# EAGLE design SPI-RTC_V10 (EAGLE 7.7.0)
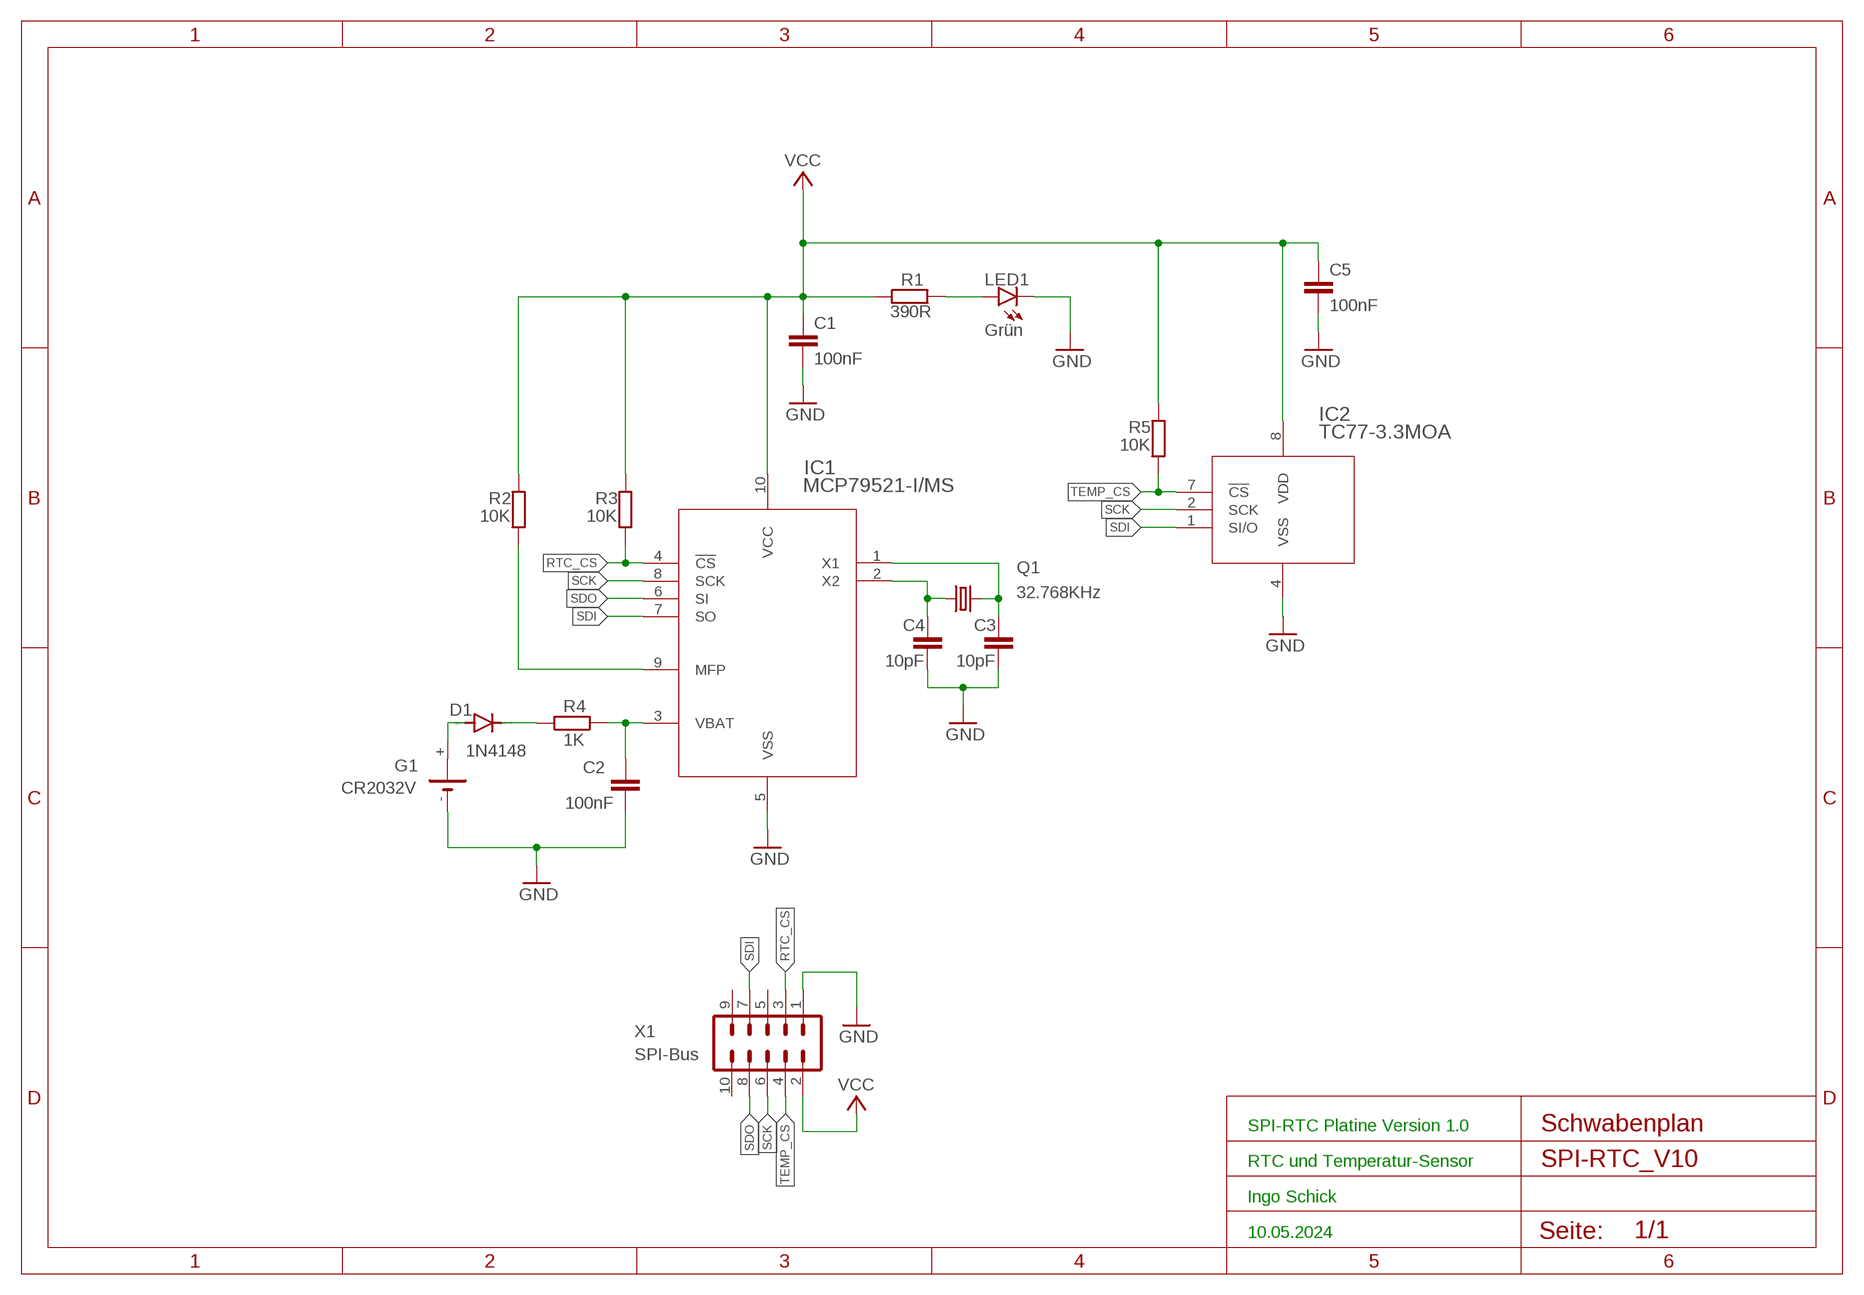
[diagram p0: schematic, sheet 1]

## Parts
C1  100nF  C-EU025-025X050  [C025-025X050]
C2  100nF  C-EU025-025X050  [C025-025X050]
C3  10pF  C-EU025-025X050  [C025-025X050]
C4  10pF  C-EU025-025X050  [C025-025X050]
C5  100nF  C-EU025-025X050  [C025-025X050]
D1  1N4148  1N4148DO35-7  [DO35-7]
G1  CR2032V  [CR2032V]
IC1  MCP79521-I/MS  [MSOP10]
IC2  TC77-3.3MOA  [SO-08]
LED1  Grün  LED3MM  [LED3MM]
Q1  32.768KHz  CRYSTALTC38H  [TC38H]
R1  390R  R-EU_0207/10  [0207/10]
R2  10K  R-EU_0207/10  [0207/10]
R3  10K  R-EU_0207/10  [0207/10]
R4  1K  R-EU_0207/10  [0207/10]
R5  10K  R-EU_0207/10  [0207/10]
X1  SPI-Bus  ML10  [ML10]

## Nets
BAT: D1.A G1.+
BAT_R: D1.C R4.2
GND: C1.2 C2.2 C3.2 C4.2 C5.2 G1.- IC1.5(VSS) IC2.4(VSS) LED1.K(C) X1.1
LED: LED1.A R1.2
MFP: IC1.9(MFP) R2.1
RTC_CS: IC1.4(!CS) R3.1 X1.3
SCK: IC1.8(SCK) IC2.2(SCK) X1.6
SDI: IC1.7(SO) IC2.1(SI/O) X1.7
SDO: IC1.6(SI) X1.8
TEMP_CS: IC2.7(!CS) R5.1 X1.4
VBAT: C2.1 IC1.3(VBAT) R4.1
VCC: C1.1 C5.1 IC1.10(VCC) IC2.8(VDD) R1.1 R2.2 R3.2 R5.2 X1.2
X1: C3.1 IC1.1(X1) Q1.2
X2: C4.1 IC1.2(X2) Q1.1
Unconnected: G1.+@1(+) X1.5 X1.9 X1.10

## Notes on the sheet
- SPI-RTC Platine Version 1.0
- RTC und Temperatur-Sensor
- Ingo Schick
- 10.05.2024

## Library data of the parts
C1-C5 = rcl:C-EU: CAPACITOR, European symbol; SPICEPREFIX: C
D1 = Schwabenplan:1N4148: 1N4148 -> Kleinsignal-Schaltdiode; FRITSCH: K-DI0001; HERSTELLER: 1N4148; MOUSER: 637-1N4148
G1 = Schwabenplan:CR2032V: Batteriehalter für CR2032; FRITSCH: K-BA0047; WUERTH: 79548211
IC1 = Schwabenplan_SPI:MCP79521: MCP79521-I/MS - SPI-Bus RTC-Baustein, EEPROM inkl. MAC-Adresse Produktinformationen: Datenblatt; HERSTELLER: MCP79521-I/MS; MOUSER: 579-MCP79521-I/MS
IC2 = Schwabenplan_SPI:TC77: TC77 - SPI-Bus Temperatur Sensor mit 13 Bit Auflösung Produktinformationen: Datenblatt; HERSTELLER: TC77-3.3MOA; MOUSER: 579-TC77-3.3MOA
LED1 = Schwabenplan_LED:LED: Schwabenplan LED
Q1 = Schwabenplan_Quarze:CRYSTAL: CRYSTAL; OC_FARNELL: unknown; OC_NEWARK: unknown
R1-R5 = rcl:R-EU_: RESISTOR, European symbol; SPICEPREFIX: R
X1 = Schwabenplan:ML10: IDE Wannenstecker 10 polig Würth: Datenblatt oder Harting: Datenblatt oder Reichelt: Datenblatt; FRITSCH: K-ST2236; HARTING: 09185106324; REICHELT: WSL 10G; WUERTH: 61201021621

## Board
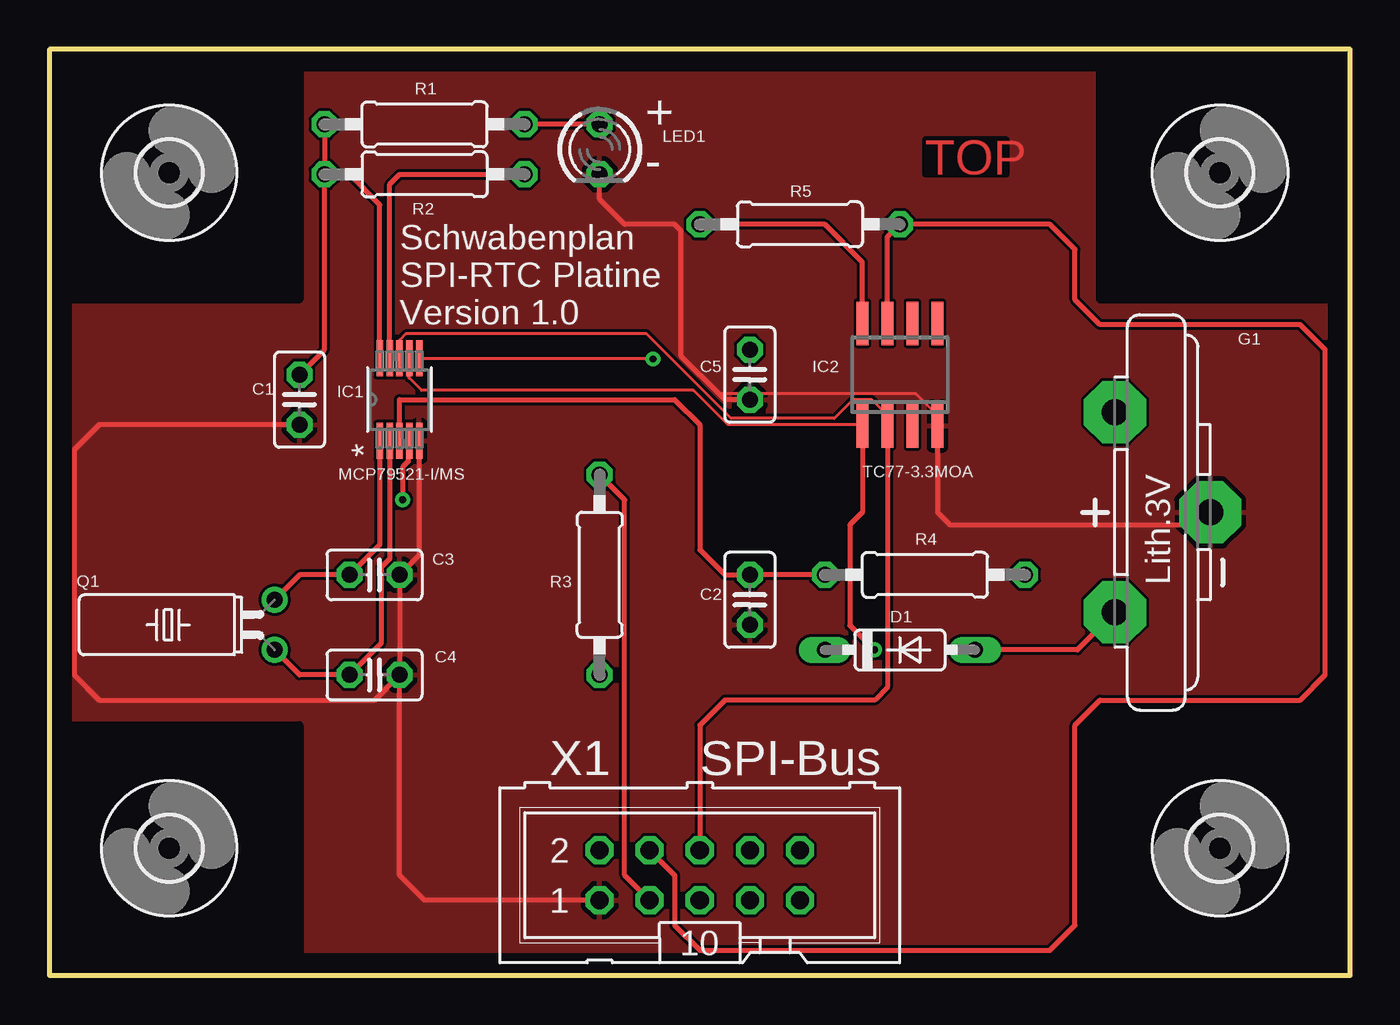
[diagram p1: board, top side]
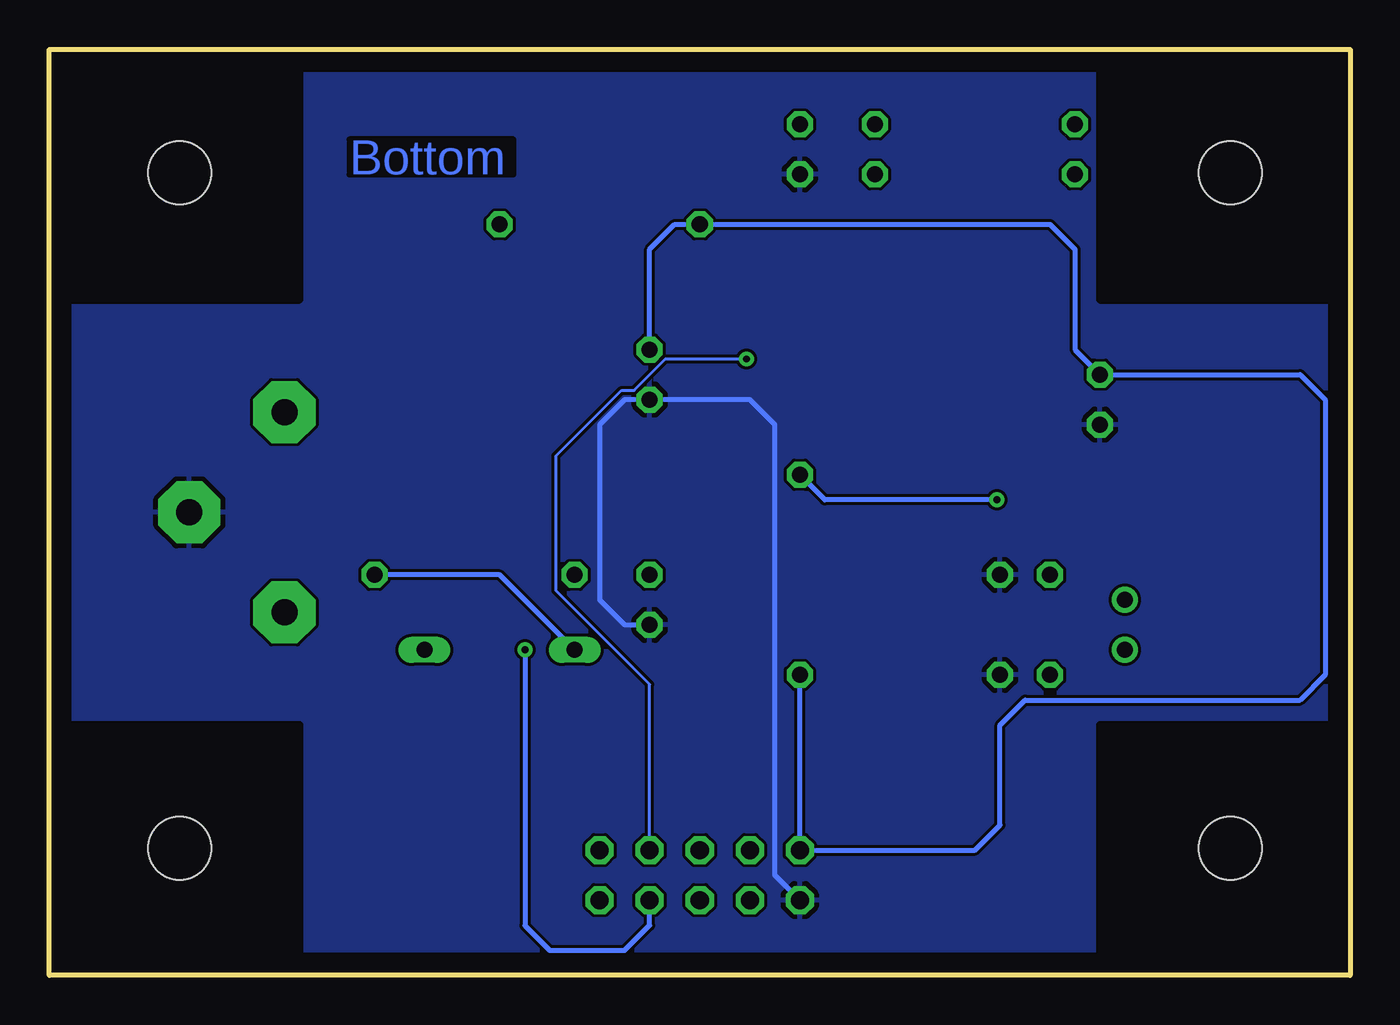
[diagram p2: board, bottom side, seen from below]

Size 66.04 x 46.99 mm. Coordinates in mm from the lower left corner, seen from the top.
Outline: 0,0 66.04,0 66.04,46.99 0,46.99 0,0
Copper layers (1*16): Top 0.035mm / dielectric 0.15mm / Bottom 0.035mm
Design rules "default": minimum track width 6mil, minimum drill 0.35mm, track to track 6mil, track to pad 6mil, pad to pad 6mil, via to via 6mil, smd to smd 6mil, copper to edge 40mil, drill to drill 6mil, minimum pad ring 10mil, minimum via ring 8mil, stop-mask expansion 4mil, vias tented up to drill 0mil, thermal gap 10mil
tRestrict: area 0,0 to 12.7,12.7; area 53.3,0 to 66,12.7; area 0,34.3 to 12.7,47; area 53.3,34.3 to 66,47
bRestrict: area 0,0 to 12.7,12.7; area 0,34.3 to 12.7,47; area 53.3,34.3 to 66,47; area 53.3,0 to 66,12.7

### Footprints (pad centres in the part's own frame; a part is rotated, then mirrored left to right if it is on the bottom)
C025-025X050 = drill 0.813 octagon: 1 -1.27,0; 2 1.27,0
DO35-7 = drill 0.813 long: A 3.81,0; C -3.81,0
CR2032V = drill 1.321 pad 3.15 octagon: + -2.54,-5.08; +@1 -2.54,5.08; - 2.286,0
MSOP10 = smd 1.829 x 0.33: 1 -2.095,1; 2 -2.095,0.5; 3 -2.095,0; 4 -2.095,-0.5; 5 -2.095,-1; 6 2.095,-1; 7 2.095,-0.5; 8 2.095,0; 9 2.095,0.5; 10 2.095,1
SO-08 = smd 0.6 x 2.2: 1 -1.905,-2.6; 2 -0.635,-2.6; 3 0.635,-2.6; 4 1.905,-2.6; 5 1.905,2.6; 6 0.635,2.6; 7 -0.635,2.6; 8 -1.905,2.6
LED3MM = drill 0.813 octagon: A -1.27,0; K 1.27,0
TC38H = drill 0.813: 1 -1.27,0; 2 1.27,0
0207/10 = drill 0.813 octagon: 1 -5.08,0; 2 5.08,0
3,2 = hole 3.2: 0,0
ML10 = drill 0.914 octagon: 1 -5.08,-1.27; 2 -5.08,1.27; 3 -2.54,-1.27; 4 -2.54,1.27; 5 0,-1.27; 6 0,1.27; 7 2.54,-1.27; 8 2.54,1.27; 9 5.08,-1.27; 10 5.08,1.27

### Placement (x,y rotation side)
C1  12.7,29.21 270 top
C2  35.56,19.05 270 top
C3  16.51,20.32 0 top
C4  16.51,15.24 0 top
C5  35.56,30.48 270 top
D1  43.18,16.51 0 top
G1  56.64,23.5 0 top
IC1  17.78,29.21 90 top
IC2  43.18,30.48 0 top
LED1  27.94,41.91 270 top
Q1  11.43,17.78 90 top
R1  19.05,43.18 0 top
R2  19.05,40.64 180 top
R3  27.94,20.32 270 top
R4  44.45,20.32 0 top
R5  38.1,38.1 180 top
U$13  [3,2]  6.09,6.44 0 top
U$14  [3,2]  59.43,6.44 0 top
U$15  [3,2]  6.09,40.73 0 top
U$16  [3,2]  59.43,40.73 0 top
X1  33.02,5.08 0 top

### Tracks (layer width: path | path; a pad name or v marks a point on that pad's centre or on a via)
BAT
  Top 0.254: G1.+ 52.2,16.51 D1.A
BAT_R
  Bottom 0.254: D1.C 43.18,20.32 R4.2
GND
  Top 0.152: IC2.4 45.09,28.42 43.97,29.53 34.13,29.53 34.05,29.45
  Top 0.254: C4.2 C3.2 18.78,21.32 IC1.5 | X1.1 19.05,3.81 17.78,5.08 C4.2 | C1.2 2.54,27.94 1.27,26.67 1.27,15.24 2.54,13.97 16.51,13.97 C4.2 | C5.2 34.29,29.21 34.05,29.45 32.08,31.42 32.08,37.77 31.75,38.1 29.21,38.1 27.94,39.37 LED1.K | IC2.4 45.09,23.5 45.72,22.86 58.29,22.86 G1.-
  Bottom 0.254: C2.2 36.83,17.78 38.1,19.05 38.1,27.94 36.83,29.21 C5.2 30.48,29.21 29.21,27.94 29.21,5.08 X1.1
  pour Bottom: 0,0 66.04,0 66.04,46.99 0,46.99
  pour Top: 0,0 66.04,0 66.04,46.99 0,46.99
LED
  Top 0.254: LED1.A R1.2
MFP
  Top 0.254: IC1.9 17.28,40.14 17.78,40.64 R2.1
RTC_CS  (via drill 0.35)
  Top 0.254: IC1.4 18.22,27.06 18.22,26.08 17.94,25.8 v17.94,24.13 | X1.3 29.21,5.08 29.21,24.13 R3.1
  Bottom 0.254: v17.94,24.13 26.67,24.13 R3.1
SCK
  Top 0.152: IC1.8 17.78,32.23 18.1,32.54 30.32,32.54 34.61,28.26 39.85,28.26 40.8,29.21 41.75,29.21 42.55,28.42 IC2.2
  Top 0.254: IC2.2 42.55,14.61 41.91,13.97 34.29,13.97 33.02,12.7 X1.6
SDI  (via drill 0.35)
  Top 0.152: IC1.7 18.26,31.27 18.26,30.32 18.89,29.69 32.7,29.69 34.45,27.94 41.27,27.94 IC2.1
  Top 0.254: IC2.1 41.27,23.5 40.64,22.86 40.64,17.76 v41.89,16.51
  Bottom 0.254: v41.89,16.51 41.89,2.52 40.64,1.27 36.83,1.27 35.56,2.54 X1.7
SDO  (via drill 0.35)
  Top 0.152: v30.64,31.27 18.89,31.27 IC1.6
  Bottom 0.152: v30.64,31.27 34.77,31.27 36.35,29.69 36.99,29.69 40.32,26.35 40.32,19.53 35.56,14.76 X1.8
TEMP_CS
  Top 0.254: IC2.7 42.55,37.47 R5.1 50.8,38.1 52.07,36.83 52.07,34.29 53.34,33.02 63.5,33.02 64.77,31.75 64.77,15.24 63.5,13.97 53.34,13.97 52.07,12.7 52.07,2.54 50.8,1.27 33.02,1.27 31.75,2.54 31.75,5.08 X1.4
VBAT
  Top 0.254: R4.1 C2.1 34.29,20.32 33.02,21.59 33.02,27.94 31.75,29.21 17.78,29.21 IC1.3
VCC
  Top 0.254: IC1.10 16.78,39.1 15.24,40.64 R2.2 | C1.1 13.97,31.75 R2.2 | R1.1 R2.2 | IC2.8 41.27,36.2 39.37,38.1 R5.2
  Bottom 0.254: C5.1 35.56,36.83 34.29,38.1 R5.2 15.24,38.1 13.97,36.83 13.97,31.75 C1.1 2.54,30.48 1.27,29.21 1.27,15.24 2.54,13.97 16.51,13.97 17.78,12.7 17.78,7.62 19.05,6.35 X1.2 R3.2
X1
  Top 0.254: Q1.2 12.7,20.32 C3.1 16.78,21.86 IC1.1
X2
  Top 0.254: Q1.1 12.7,15.24 C4.1 16.84,16.84 16.84,20.71 17.28,21.15 IC1.2

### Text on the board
Top: TOP
Bottom: Bottom
tNames: + | - | Schwabenplan / SPI-RTC Platine / Version 1.0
